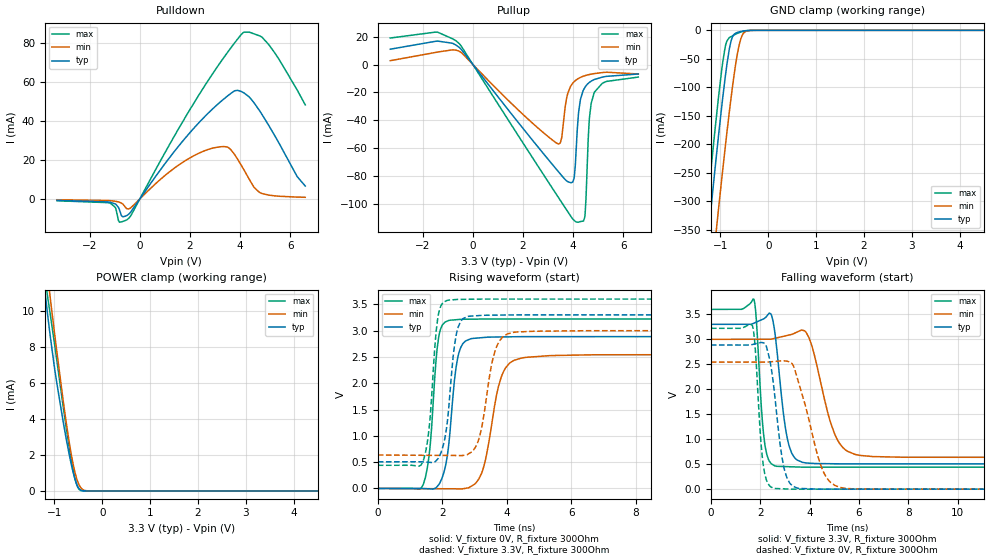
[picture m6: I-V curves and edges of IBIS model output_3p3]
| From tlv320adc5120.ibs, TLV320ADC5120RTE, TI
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|   output_3p3 Model
[Model]   output_3p3
Model_type   3-state
Polarity   Non-Inverting
Vmeas = 1.65
Vref = 0
Cref = 2pF
Rref = 100000
|   typ   min   max
C_comp   2.453pF   2.442pF   2.453pF
| Where Nom  PVT is Nominal Process, 3.3V, 27C
|   Fast PVT is Strong Process,  3.6V, -40C
|   Slow PVT is Weak Process,   3.0V, 150C
[Voltage Range]   3.3   3   3.6
|Junction Temperature
[Temperature Range]   27   150   -40
[Pullup Reference]   3.3   3   3.6
[Pulldown Reference]   -0   -0   0
[Power Clamp Reference]   3.3   3   3.6
[GND Clamp Reference]   0   0   0
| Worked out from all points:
|   slope of the pulldown table from 0 to 0.495 V, typ, clamps not added: 54.4 ohm
|   slope of the pullup table from 0 to 0.495 V, typ, clamps not added: 43 ohm
|   GND clamp passes 1 mA (typ) near -0.51 V on its own axis
|   POWER clamp passes 1 mA (typ) near -0.60 V on its own axis
|   falling waveform, V_fixture 3.3V, R_fixture 300Ohm: 20-80 % time 394ps typ, 741ps min, 248ps max; typ from 3.3 V to 0.506 V
|   rising waveform, V_fixture 0V, R_fixture 300Ohm: 20-80 % time 286ps typ, 463ps min, 235ps max; typ from 0 V to 2.89 V
|   rising waveform, V_fixture 3.3V, R_fixture 300Ohm: 20-80 % time 273ps typ, 393ps min, 231ps max; typ from 0.506 V to 3.3 V
|   falling waveform, V_fixture 0V, R_fixture 300Ohm: 20-80 % time 423ps typ, 819ps min, 252ps max; typ from 2.89 V to 0 V
[Pulldown]
|   Voltage   I(typ)   I(min)   I(max)
-3.3V     -787.2uA   -457.1uA   -983.8uA
-1.251V   -1.601mA   -877.8uA   -1.981mA
-983.4mV  -2.618mA   -1.235mA   -4.346mA
-815.1mV  -5.606mA   -1.733mA   -11.98mA
-676.5mV  -9.238mA   -2.726mA   -11.58mA
-438.9mV  -7.81mA    -5.172mA   -9.929mA
2.373V    39.34mA    23.54mA    53.69mA
3.482V    52.66mA    26.65mA    74.92mA
3.897V    55.72mA    20.43mA    82.01mA
4.155V    54.38mA    14.86mA    85.59mA
4.877V    43.25mA    2.736mA    82.97mA
6.6V      6.576mA    807.3uA    48.26mA
[GND Clamp]
|   Voltage   I(typ)   I(min)   I(max)
-3.3V     -2.212A    -2.319A    -2.156A
-1.34V    -433.7mA   -561.8mA   -365.6mA
-1.3V     -399.7mA   -528.3mA   -331.3mA
-1.231V   -340.8mA   -470mA     -272mA
-1.102V   -234.4mA   -363.8mA   -165.6mA
-1.043V   -187.1mA   -316mA     -119.3mA
-904.2mV  -85.05mA   -208.5mA   -30.84mA
-785.4mV  -21.13mA   -123.5mA   -11.39mA
-656.7mV  -4.076mA   -46.57mA   -5.711mA
-547.8mV  -1.572mA   -9.26mA    -2.381mA
-379.5mV  -89.03uA   -265.2uA   -154.4uA
6.6V      0A         0A         0A
[Pullup]
|   Voltage   I(typ)   I(min)   I(max)
-3.3V     11mA       2.749mA    19.02mA
-537.9mV  12.19mA    9.482mA    14.9mA
3.422V    -77.12mA   -56.99mA   -95.67mA
3.759V    -83.76mA   -22.56mA   -104.9mA
3.986V    -84.25mA   -13.35mA   -110.9mA
4.085V    -72.49mA   -11.56mA   -112.5mA
4.165V    -46.6mA    -10.51mA   -113.1mA
4.283V    -25.8mA    -9.313mA   -112.7mA
4.462V    -16.62mA   -8.058mA   -109.7mA
4.64V     -12.94mA   -7.194mA   -40.63mA
4.838V    -10.81mA   -6.517mA   -20.24mA
6.6V      -6.788mA   -6.785mA   -9.012mA
[POWER Clamp]
|   Voltage   I(typ)   I(min)   I(max)
-3.3V     67.3mA     63.88mA    75.21mA
-1.241V   12.15mA    14.24mA    12.75mA
-1.142V   9.839mA    12mA       10.84mA
-1.092V   8.755mA    10.89mA    9.949mA
-963.6mV  6.261mA    8.079mA    7.554mA
-815.1mV  3.84mA     5.014mA    4.678mA
-686.4mV  1.989mA    2.662mA    2.368mA
-557.7mV  558.4uA    914.7uA    571.5uA
-508.2mV  227.6uA    491uA      186.2uA
-448.8mV  46.37uA    181.8uA    23.04uA
-260.7mV  352.3nA    1.536uA    0A
6.6V      0A         0A         0A
[Ramp]
R_load = 300
|   typ   min   max
dV/dt_r   1.73193/2.84224e-10   1.5269/4.59772e-10   1.93281/2.33403e-10
dV/dt_f   1.67613/3.92838e-10   1.41861/7.40033e-10   1.89609/2.47348e-10
[Falling Waveform]
V_fixture = 3.3V
V_fixture_min = 3V
V_fixture_max = 3.6V
R_fixture = 300Ohm
C_fixture = 0F
|   Time   V(typ)   V(min)   V(max)
0s        3.3V       3V         3.6V
1.741ns   3.323V     3.002V     3.804V
2.171ns   3.42V      3.002V     950.7mV
2.589ns   3.145V     3.02V      466.6mV
3.108ns   987.4mV    3.08V      450.4mV
3.71ns    537.2mV    3.182V     440.7mV
4.067ns   518mV      2.906V     440.5mV
5.013ns   508.7mV    1.104V     440.5mV
5.83ns    507.6mV    697.4mV    440.4mV
20ns      506.5mV    635.6mV    439.8mV
[Rising Waveform]
V_fixture = 0V
V_fixture_min = 0V
V_fixture_max = 0V
R_fixture = 300Ohm
C_fixture = 0F
|   Time   V(typ)   V(min)   V(max)
0s        -3.013nV   10.52nV    -7.288nV
1.404ns   -1.181mV   -4.258mV   71.15mV
1.614ns   -8.732mV   -4.892mV   765.9mV
1.881ns   66.1mV     -5.703mV   2.855V
2.191ns   796.9mV    -6.643mV   3.192V
2.626ns   2.744V     -7.528mV   3.216V
3.237ns   2.867V     324.8mV    3.22V
3.861ns   2.88V      2.174V     3.221V
4.462ns   2.886V     2.48V      3.221V
20ns      2.887V     2.545V     3.221V
[Rising Waveform]
V_fixture = 3.3V
V_fixture_min = 3V
V_fixture_max = 3.6V
R_fixture = 300Ohm
C_fixture = 0F
|   Time   V(typ)   V(min)   V(max)
0s        506.5mV    635.6mV    439.8mV
1.397ns   505.3mV    630.1mV    507.6mV
1.6ns     496.5mV    629.3mV    1.207V
1.851ns   556.6mV    628.3mV    3.209V
2.152ns   1.253V     627.1mV    3.575V
2.568ns   3.175V     625.5mV    3.595V
3.089ns   3.284V     865.1mV    3.598V
3.643ns   3.295V     2.633V     3.6V
4.179ns   3.298V     2.965V     3.6V
20ns      3.3V       3V         3.6V
[Falling Waveform]
|Gnd
V_fixture = 0V
V_fixture_min = 0V
V_fixture_max = 0V
R_fixture = 300Ohm
C_fixture = 0F
|   Time   V(typ)   V(min)   V(max)
0s        2.887V     2.545V     3.221V
1.681ns   2.897V     2.544V     3.275V
1.794ns   2.91V      2.544V     2.837V
2.115ns   2.932V     2.544V     505.1mV
2.532ns   2.11V      2.555V     20.77mV
2.884ns   627.3mV    2.571V     7.651mV
3.18ns    132.6mV    2.544V     1.733mV
4.522ns   685.2uV    387.4mV    453.9uV
5.251ns   652.9uV    33.43mV    432.5uV
20ns      2.953nV    -56.16nV   1.011nV
